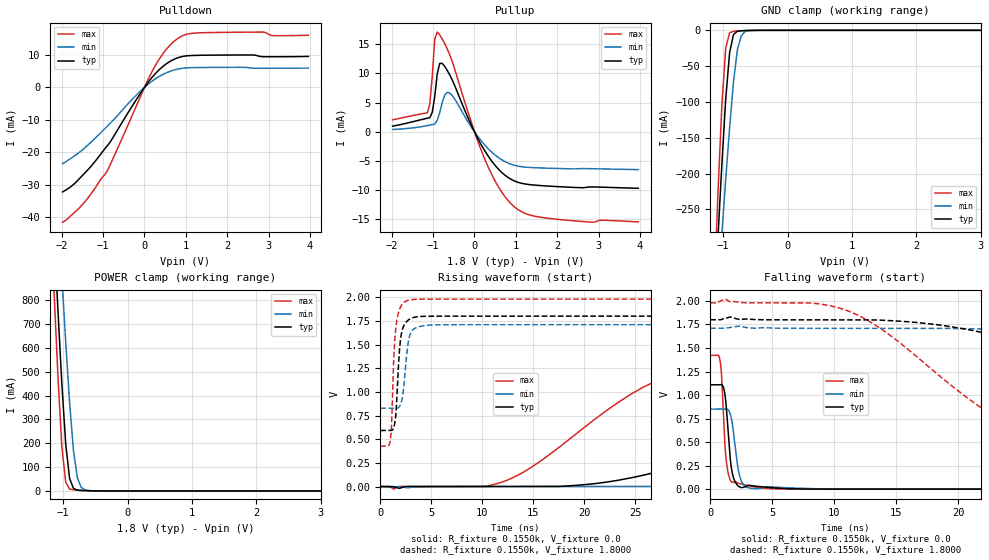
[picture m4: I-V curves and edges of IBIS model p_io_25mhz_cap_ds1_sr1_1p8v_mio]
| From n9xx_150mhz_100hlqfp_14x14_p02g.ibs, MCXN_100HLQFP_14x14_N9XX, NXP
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[Model] p_io_25mhz_cap_ds1_sr1_1p8v_mio
|   Model p_io_25mhz_cap_ds1_sr1_1p8v_mio
| This model was characterised for following simulation conditions:
| External (pad) voltage:
|   - Typ: 1.8V,   - Min: 1.71V,   - Max: 1.98V
| Library cells for typ/min/max conditions are connected as defined below:
|  pad - External Pad
|  ipp_do_lv - Core Input
|  ipp_obe_lv - Output Buffer Enable
|  IOGC - NC
|  REFH3V3 - REFH3V3
|  REFL3V3 - REFL3V3
|  ZI - NC
|  abut_ncal_vddio[1] - vssio vddio vddio
|  abut_ncal_vddio[2] - vddio vddio vssio
|  abut_ncal_vddio[3] - vddio
|  abut_ncal_vddio[4] - vssio vddio vddio
|  abut_ncal_vddio[5] - vddio vddio vssio
|  abut_ncal_vddio[6] - vddio
|  abut_pcal_vddio[1] - vssio
|  abut_pcal_vddio[2] - vddio vssio vddio
|  abut_pcal_vddio[3] - vssio
|  abut_pcal_vddio[4] - vssio
|  abut_pcal_vddio[5] - vddio vssio vddio
|  abut_pcal_vddio[6] - vssio
|  ipp_do_1p8v - ipp_do_1p8v
|  ipp_dse_lv - vdd_lv
|  ipp_eftd_lv - NC
|  ipp_ina_mux_vddio - NC
|  ipp_ina_mux_vddio[0] - NC
|  ipp_ina_mux_vddio[1] - NC
|  ipp_ina_r0_vddio - NC
|  ipp_ina_r0a_vddio - NC
|  ipp_ina_r0b_vddio - NC
|  ipp_ina_r0c_vddio - NC
|  ipp_ina_r0d_vddio - NC
|  ipp_ina_r0e_vddio - NC
|  ipp_ina_r0f_vddio - NC
|  ipp_ina_r300_vddio - NC
|  ipp_ina_r300a_vddio - NC
|  ipp_ina_r300b_vddio - NC
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Model_type I/O
Polarity   Non-Inverting
Enable   Active-High
Vinl =   0.5400V
Vinh =   1.2600V
Vmeas =  0.9000V
Cref =   30.0000pF
Rref =   1.0000M
Vref =   1.8000V
C_comp   1.3068pF   1.2541pF   1.3694pF
|C_comp_pullup   0.5695pF   0.5987pF   0.5427pF
|C_comp_pulldown   0.6505pF   0.6823pF   0.6255pF
[Model Spec]
| variable   typ   min   max
Vinh   1.2600V   1.1970V   1.3860V
Vinl   0.5400V   0.5130V   0.5940V
[Temperature Range]   25.0000   0.1250k   -40.0000
[Voltage Range]   1.8000V   1.7100V   1.9800V
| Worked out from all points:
|   slope of the pulldown table from 0 to 0.27 V, typ, clamps not added: 62.4 ohm
|   slope of the pullup table from 0 to 0.27 V, typ, clamps not added: 77.5 ohm
|   GND clamp passes 1 mA (typ) near -0.76 V on its own axis
|   POWER clamp passes 1 mA (typ) near -0.63 V on its own axis
|   rising waveform, R_fixture 0.1550k, V_fixture 0.0: 20-80 % time 23.2ns typ, 43.7ns min, 11.7ns max; typ from 0 V to 1.11 V
|   rising waveform, R_fixture 0.1550k, V_fixture 1.8000: 20-80 % time 420ps typ, 510ps min, 382ps max; typ from 0.592 V to 1.8 V
|   falling waveform, R_fixture 0.1550k, V_fixture 0.0: 20-80 % time 425ps typ, 523ps min, 367ps max; typ from 1.11 V to 0 V
|   falling waveform, R_fixture 0.1550k, V_fixture 1.8000: 20-80 % time 18.9ns typ, 36.9ns min, 9.36ns max; typ from 1.8 V to 0.592 V
[Pulldown]
|Voltage   I(typ)   I(min)   I(max)
-1.98V    -32.19mA   -23.51mA   -41.49mA
-1.74V    -30.15mA   -21.53mA   -39.06mA
-1.44V    -26.34mA   -18.56mA   -35.19mA
-900mV    -18.01mA   -11.95mA   -25.73mA
180mV     3.037mA    1.878mA    4.81mA
480mV     6.798mA    4.207mA    10.95mA
780mV     8.998mA    5.569mA    14.83mA
1.02V     9.704mA    6.009mA    16.35mA
1.38V     9.882mA    6.119mA    16.81mA
2.88V     9.44mA     5.884mA    17mA
3.12V     9.433mA    5.887mA    15.93mA
3.96V     9.528mA    5.94mA     16.05mA
[Pullup]
|Voltage   I(typ)   I(min)   I(max)
-1.98V    966.2uA    399.3uA    2.044mA
-1.14V    2.321mA    1.063mA    3.243mA
-1.08V    2.416mA    1.15mA     4.764mA
-1.02V    3.358mA    1.24mA     9.557mA
-960mV    6.04mA     1.332mA    15.9mA
-900mV    9.92mA     1.974mA    17.06mA
-780mV    11.71mA    5.034mA    15.89mA
-600mV    9.758mA    6.666mA    13.21mA
240mV     -3.146mA   -2.189mA   -4.533mA
900mV     -8.184mA   -5.592mA   -12.42mA
1.68V     -9.239mA   -6.201mA   -14.7mA
3.96V     -9.667mA   -6.471mA   -15.41mA
[GND_clamp]
|Voltage   I(typ)   I(min)   I(max)
-1.98V    -2A        -1.65A     -2.499A
-1.14V    -394mA     -441.5mA   -363.8mA
-1.08V    -288.3mA   -361.7mA   -226.5mA
-1.02V    -187.2mA   -283.6mA   -103.8mA
-960mV    -95.64mA   -207.9mA   -24.71mA
-900mV    -31.47mA   -136.2mA   -3.431mA
-840mV    -6.005mA   -72.18mA   -1.326mA
-780mV    -1.297mA   -27.91mA   -902.8uA
-720mV    -576.7uA   -7.632mA   -619.4uA
-660mV    -346.6uA   -1.808mA   -391.2uA
-420mV    -13.9uA    -31.16uA   -8.588uA
3.96V     0A         0A         0A
[POWER_clamp]
|Voltage   I(typ)   I(min)   I(max)
-1.98V    5.618A     5.349A     6.084A
-1.14V    1.071A     1.443A     829.6mA
-1.08V    754.2mA    1.168A     476.4mA
-1.02V    449mA      895.6mA    184.6mA
-960mV    195.8mA    625.5mA    36.79mA
-900mV    52.44mA    371.1mA    7.808mA
-840mV    10.74mA    170.2mA    4.435mA
-780mV    3.619mA    56.22mA    3.182mA
-720mV    2.074mA    15.04mA    2.195mA
-660mV    1.306mA    4.299mA    1.376mA
-360mV    5.079uA    27.62uA    1.341uA
3.96V     0A         0A         0A
[Ramp]
| variable   typ   min   max
dV/dt_r  0.6652/23.2038n   0.5082/43.6884n   0.8531/11.7389n
dV/dt_f  0.7249/18.8624n   0.5286/36.9329n   0.9321/9.3582n
R_load = 0.1550k
[Rising Waveform]
R_fixture= 0.1550k
V_fixture= 0.0
V_fixture_min= 0.0
V_fixture_max= 0.0
|time   V(typ)   V(min)   V(max)
0s        440.2pV    137.5nV    11.95pV
11.82ns   -24.85uV   -7.732uV   42.51mV
20.19ns   21.14mV    64.24uV    640.6mV
27.31ns   157.8mV    2.456mV    1.124V
40.83ns   594.8mV    73.28mV    1.345V
49.85ns   838.7mV    171.5mV    1.384V
59.83ns   964.5mV    305.7mV    1.403V
81.21ns   1.058V     583.4mV    1.418V
102.6ns   1.089V     722.9mV    1.421V
235ns     1.109V     847mV      1.422V
[Rising Waveform]
R_fixture= 0.1550k
V_fixture= 1.8000
V_fixture_min= 1.7100
V_fixture_max= 1.9800
|time   V(typ)   V(min)   V(max)
0s        591.8mV    826.8mV    426.4mV
1.012ns   591.5mV    826.8mV    509.8mV
1.114ns   592.2mV    826.8mV    670.7mV
1.388ns   651.6mV    826.8mV    1.488V
1.724ns   1.154V     829.5mV    1.812V
1.915ns   1.482V     850.7mV    1.879V
2.168ns   1.659V     941.7mV    1.928V
2.753ns   1.759V     1.53V      1.968V
3.313ns   1.787V     1.666V     1.976V
235ns     1.8V       1.71V      1.98V
[Falling Waveform]
R_fixture= 0.1550k
V_fixture= 0.0
V_fixture_min= 0.0
V_fixture_max= 0.0
|time   V(typ)   V(min)   V(max)
0s        1.109V     850.6mV    1.422V
794.6ps   1.11V      850.5mV    1.362V
909.3ps   1.111V     850.5mV    1.205V
1.227ns   959.4mV    853.5mV    387.5mV
1.599ns   336.8mV    801.8mV    99.55mV
1.928ns   99.28mV    539.7mV    75.28mV
2.248ns   34.8mV     214.7mV    64.77mV
2.57ns    17.71mV    69.67mV    52.17mV
4.789ns   17.25mV    25.65mV    5.484mV
235ns     91.32nV    1.858uV    12.18nV
[Falling Waveform]
R_fixture= 0.1550k
V_fixture= 1.8000
V_fixture_min= 1.7100
V_fixture_max= 1.9800
|time   V(typ)   V(min)   V(max)
0s        1.8V       1.71V      1.98V
10.5ns    1.8V       1.71V      1.921V
13.83ns   1.796V     1.71V      1.698V
23.71ns   1.611V     1.696V     723.5mV
35.02ns   1.141V     1.605V     503.8mV
41.81ns   885.6mV    1.513V     470.7mV
49.81ns   752.2mV    1.382V     450.9mV
67.67ns   653mV      1.092V     433.9mV
88.45ns   615.7mV    947.1mV    428.4mV
235ns     591.8mV    829mV      426.4mV
